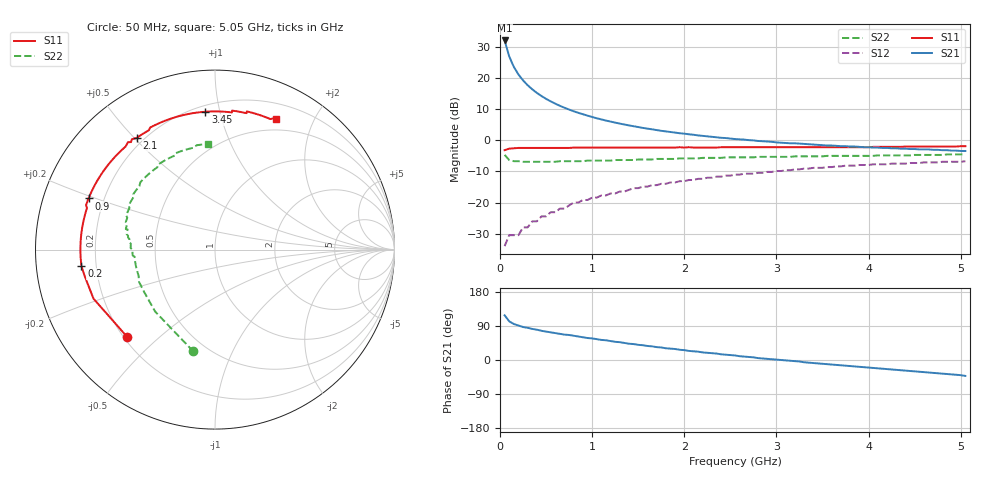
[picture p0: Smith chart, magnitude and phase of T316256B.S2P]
!AT-31625
!S-PARAMETERS at Vce=6.0 V  Ic=100 mA.  LAST UPDATED 08-05-96
# ghz s ma r 50
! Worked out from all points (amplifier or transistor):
!   101 points, 50 MHz to 5.05 GHz, reference 50 ohm
!   highest |S21| = 31.9 dB at 50 MHz (marker M1)
!   |S21| within 3 dB of that: start of sweep to 79.26 MHz
!   unconditionally stable (mu >= 1): 481.7 MHz to 1.544 GHz; 1.556 GHz to 1.631 GHz
!   at 850 MHz: K = 1.03, MAG = 13.4 dB, |S12| = -20.0 dB
!   at 2.55 GHz: K = 0.95, MSG = 5.7 dB, |S12| = -11.1 dB
!   at 5.05 GHz: K = 0.93, MSG = 1.6 dB, |S12| = -6.7 dB
!   S11 on the Smith chart (normalised r, x): 50 MHz: 0.21, -0.40; 200 MHz: 0.14, -0.06; 900 MHz: 0.14, +0.19; 2.1 GHz: 0.17, +0.51; 3.45 GHz: 0.24, +0.90; 5.05 GHz: 0.37, +1.50
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0.05  0.69 -135.0  39.55 118.0  0.02 42.0  0.58 -102.0
0.1  0.73 -158.0  21.92 102.0  0.03 41.0  0.48 -134.0
0.15  0.74 -168.0  14.92 95.0  0.03 45.0  0.46 -149.0
0.2  0.75 -173.0  11.28 91.0  0.03 49.0  0.46 -157.0
0.25  0.75 -177.0  9.07 87.0  0.04 53.0  0.45 -161.0
0.3  0.75 180.0  7.58 85.0  0.04 56.0  0.45 -165.0
0.35  0.75 177.0  6.52 82.0  0.05 58.0  0.45 -167.0
0.4  0.75 175.0  5.71 80.0  0.05 59.0  0.45 -169.0
0.45  0.75 173.0  5.09 77.0  0.06 60.0  0.45 -171.0
0.55  0.75 169.0  4.18 73.0  0.07 62.0  0.45 -174.0
0.65  0.75 165.0  3.55 69.0  0.08 62.0  0.46 -176.0
0.8  0.76 161.0  2.9 64.0  0.1 62.0  0.46 -179.0
0.9  0.76 158.0  2.6 60.0  0.11 61.0  0.46 180.0
1.05  0.76 153.0  2.24 55.0  0.12 60.0  0.47 178.0
1.25  0.76 148.0  1.91 48.0  0.14 58.0  0.48 175.0
1.75  0.76 134.0  1.41 33.0  0.2 51.0  0.5 169.0
2.1  0.76 125.0  1.22 23.0  0.23 45.0  0.51 165.0
2.55  0.77 114.0  1.04 12.0  0.28 37.0  0.53 158.0
3.4  0.77 95.0  0.85 -8.0  0.36 22.0  0.55 142.0
3.45  0.77 94.0  0.84 -9.0  0.36 21.0  0.55 141.0
4.25  0.78 79.0  0.74 -25.0  0.42 4.0  0.57 119.0
5.05  0.8 65.0  0.67 -42.0  0.46 -13.0  0.59 94.0
